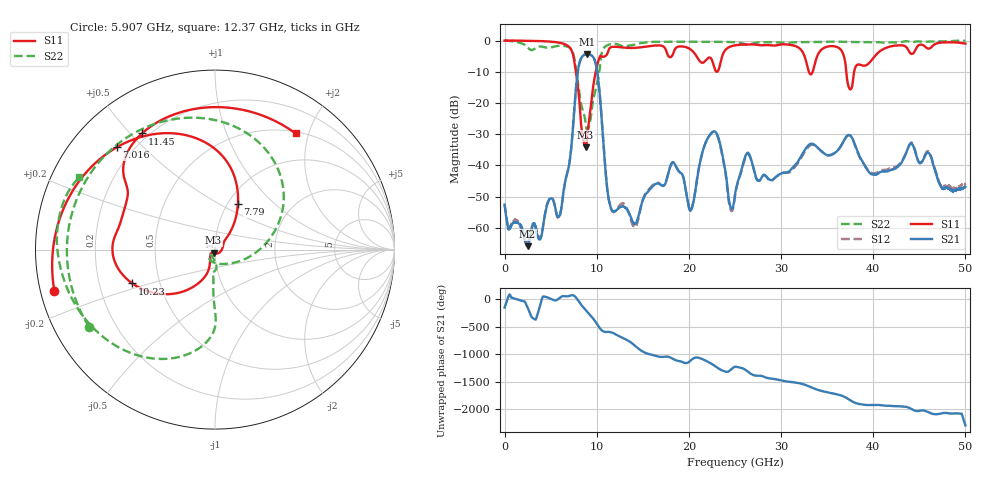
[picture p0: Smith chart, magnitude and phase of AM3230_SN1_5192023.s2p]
!Agilent Technologies,E8364B,MY43040894,A.07.50.67
!Agilent E8364B: A.07.50.67
!Date: Friday, May 19, 2023 06:57:50
!Correction: S11(Full 2 Port(1,2))
!S21(Full 2 Port(1,2))
!S12(Full 2 Port(1,2))
!S22(Full 2 Port(1,2))
!S2P File: Measurements: S11, S21, S12, S22:
# Hz S  dB  R 50
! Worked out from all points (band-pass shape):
!   6401 points, 10 MHz to 50 GHz, reference 50 ohm
!   highest |S21| = -4.29 dB at 8.993 GHz (marker M1); lowest = -65.8 dB at 2.502 GHz (marker M2)
!   |S21| within 3 dB of the highest: 8.117 GHz to 9.888 GHz (1.771 GHz wide, 19.7 % of centre)
!   lowest |S11| = -34.2 dB at 8.797 GHz (marker M3), VSWR 1.04, Z = 49.2 - j1.76 ohm
!   |S11| at or under -10 dB: 7.743 GHz to 9.897 GHz (2.153 GHz wide, 24.4 % of centre); 33.01 GHz to 33.43 GHz (418.3 MHz wide, 1.26 % of centre); 37.08 GHz to 37.93 GHz (850.2 MHz wide, 2.27 % of centre)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
!   |S22| runs from -28.6 to 0.0 dB; largest |S21 - S12| = 0.0092
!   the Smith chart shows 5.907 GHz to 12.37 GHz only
!   S11 on the Smith chart (normalised r, x): 5.907 GHz: 0.04, -0.13; 7.016 GHz: 0.14, +0.42; 7.79 GHz: 1.12, +0.61; 10.23 GHz: 0.35, -0.17; 11.45 GHz: 0.17, +0.54; 12.37 GHz: 0.53, +1.79
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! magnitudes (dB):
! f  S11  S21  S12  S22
! 10 MHz  0.0  -52.5  -52.5  0.0
! 2.502 GHz  -0.1  -65.8  -64.7  -2.2
! 5.907 GHz  -0.7  -56.4  -56.7  -1.7
! 7.016 GHz  -2.0  -39.7  -39.7  -2.2
! 7.79 GHz  -11.0  -14.1  -14.2  -9.9
! 8.344 GHz  -27.9  -5.5  -5.6  -20.8
! 8.797 GHz  -34.2  -4.4  -4.4  -26.4
! 8.993 GHz  -30.0  -4.3  -4.3  -28.6
! 10.23 GHz  -6.1  -14.0  -14.1  -10.9
! 11.45 GHz  -2.3  -52.6  -52.8  -1.2
! 12.37 GHz  -2.1  -53.7  -53.3  -1.3
! 16.68 GHz  -1.6  -45.8  -45.5  -0.4
! 18.38 GHz  -3.5  -39.2  -39.1  -0.4
! 20.24 GHz  -3.0  -54.2  -54.2  -0.4
! 22.75 GHz  -8.6  -29.1  -29.2  -0.4
! 25 GHz  -1.5  -49.4  -49.5  -0.5
! 26.32 GHz  -1.3  -36.0  -36.4  -1.3
! 28.97 GHz  -1.6  -44.7  -44.9  -0.6
! 33.34 GHz  -10.6  -33.0  -33.4  -0.5
! 41.67 GHz  -2.1  -41.8  -41.1  -0.6
! 44.14 GHz  -4.3  -33.0  -32.6  -0.5
! 50 GHz  -1.0  -46.8  -46.0  0.0
